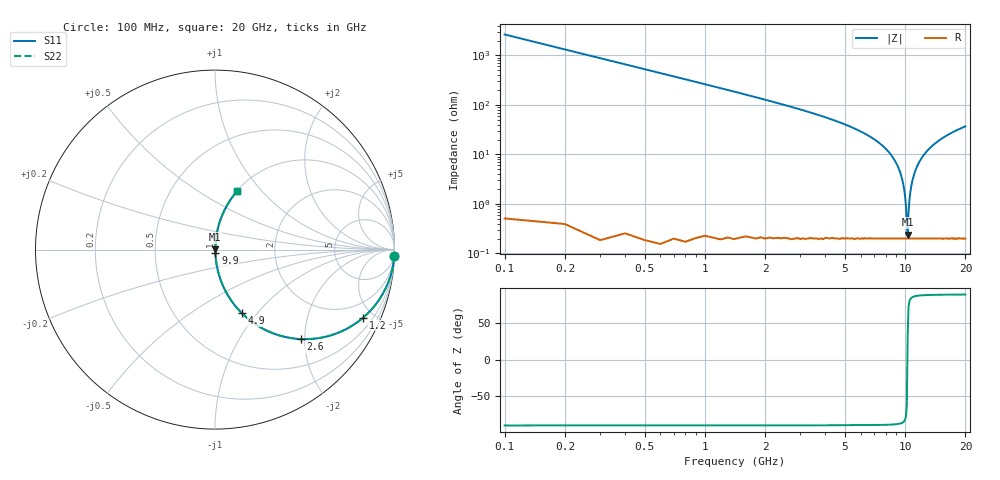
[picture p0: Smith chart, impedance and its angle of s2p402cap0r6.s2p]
! AVX Thin Film Operation		Date: April 2003
! Description: Accu-P® Series, Thin Film, SMD, RF Capacitor
! Part Number: 04021J0R6ABS
! 50 MHz  -  20 GHz
! Serial Measurements
# hz S db R 50
!	S11		S21		S12		S22
!	dB	Phase	dB	Phase	dB	Phase	dB	Phase
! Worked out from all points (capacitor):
!   200 points, 100 MHz to 20 GHz, reference 50 ohm
!   read as one part in series: C = 600 fF near 200 MHz
!   lowest |Z| = 241 mohm at 10.3 GHz (marker M1)
!   series resonance near 10.27 GHz, so ESL is about 400 pH
!   S11 on the Smith chart (normalised r, x): 100 MHz: 1, -53; 1.2 GHz: 1.00, -4.36; 2.6 GHz: 1.00, -1.91; 4.9 GHz: 1.00, -0.84; 9.9 GHz: 1.00, -0.04; 20 GHz: 1.00, +0.74
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1e8  -0.01 -2.2  -28.48 87.8  -28.48 87.8  -0.01 -2.2
2e8  -0.02 -4.3  -22.47 85.7  -22.47 85.7  -0.02 -4.3
4e8  -0.10 -8.6  -16.52 81.4  -16.52 81.4  -0.10 -8.6
7e8  -0.30 -14.8  -11.83 75.1  -11.83 75.1  -0.30 -14.8
1.2e9  -0.83 -24.6  -7.60 65.3  -7.60 65.3  -0.83 -24.6
2.6e9  -3.23 -46.3  -2.82 43.6  -2.82 43.6  -3.23 -46.3
3.5e9  -5.10 -56.1  -1.62 33.8  -1.62 33.8  -5.10 -56.1
4.9e9  -8.29 -67.1  -0.71 22.6  -0.71 22.6  -8.29 -67.1
6.8e9  -13.40 -77.1  -0.22 12.3  -0.22 12.3  -13.40 -77.1
8.9e9  -22.61 -84.2  -0.04 4.2  -0.04 4.2  -22.61 -84.2
9.5e9  -27.87 -84.9  -0.02 2.3  -0.02 2.3  -27.87 -84.9
9.9e9  -34.34 -82.9  -0.02 1.1  -0.02 1.1  -34.34 -82.9
1.01e10  -40.92 -76.7  -0.02 0.5  -0.02 0.5  -40.92 -76.7
1.03e10  -52.39 33.6  -0.02 -0.1  -0.02 -0.1  -52.39 33.6
1.04e10  -43.58 72.1  -0.02 -0.4  -0.02 -0.4  -43.58 72.1
1.05e10  -38.85 79.3  -0.02 -0.6  -0.02 -0.6  -38.85 79.3
1.07e10  -33.53 83.4  -0.02 -1.2  -0.02 -1.2  -33.53 83.4
1.1e10  -29.05 84.7  -0.02 -2.0  -0.02 -2.0  -29.05 84.7
1.19e10  -22.40 84.2  -0.04 -4.3  -0.04 -4.3  -22.40 84.2
1.34e10  -17.25 81.3  -0.10 -7.9  -0.10 -7.9  -17.25 81.3
1.67e10  -11.97 75.0  -0.30 -14.6  -0.30 -14.6  -11.97 75.0
2e10  -9.21 69.4  -0.57 -20.3  -0.57 -20.3  -9.21 69.4
